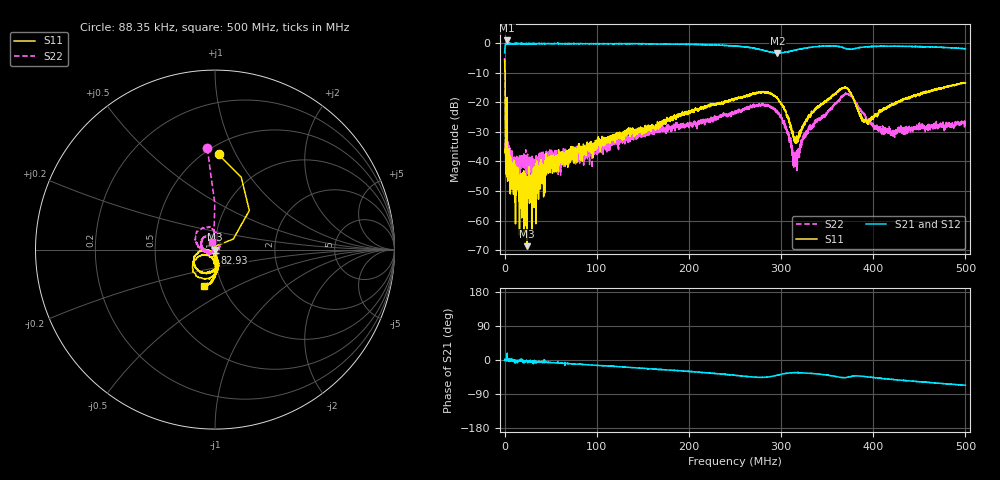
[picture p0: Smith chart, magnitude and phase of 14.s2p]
#  HZ  S  MA  R  50.00
! Rohde & Schwarz Vector Network Analyzer
! Rohde-Schwarz,ZNL6-2Port,1323001206101378,1.50.1.34-21.10.1.104
! Created: UTC 2/26/2024, 3:35:12 AM
! freq[Hz]  mag:S11  ang:S11  mag:S21  ang:S21  mag:S12  ang:S12  mag:S22  ang:S22
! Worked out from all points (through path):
!   5999 points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, 88.35 kHz to 500 MHz, reference 50 ohm
!   highest |S21| = 0.99 dB at 2.922 MHz (marker M1); lowest = -3.3 dB at 296.1 MHz (marker M2)
!   group delay of S21, straight-line fit = 332 ps
!   lowest |S11| = -68.7 dB at 24.34 MHz (marker M3), VSWR 1.00, Z = 50 - j0.0362 ohm
!   |S11| at or under -10 dB: 546.7 kHz to end of sweep
!   |S22| runs from -46.1 to -5.0 dB; largest |S21 - S12| = 0.35
!   S11 on the Smith chart (normalised r, x): 88.35 kHz: 0.58, +0.85; 82.93 MHz: 1.00, -0.04; 500 MHz: 0.82, -0.35
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88346.39  0.5305 87.8  0.6912 -1.2  0.6993 3.5  0.5653 94.3
2922124  0.1213 84.8  1.121 17.9  0.8209 7.2  0.1112 139.5
3838934  0.00873 145.6  0.9937 1.9  0.976 -2.9  0.01575 140.8
1.050665e7  0.005524 113.0  0.9865 -5.0  0.9874 1.7  0.009085 143.3
1.709101e7  0.002003 -136.5  0.9916 -1.8  0.988 -2.9  0.01002 166.5
2.434215e7  0.0003676 -79.9  0.9827 -4.1  0.9919 -2.5  0.01065 -176.5
4.634559e7  0.01126 -98.2  0.9913 -6.3  0.9911 -6.7  0.01222 -161.7
8.293466e7  0.01819 -84.7  0.9914 -11.5  0.9832 -12.3  0.0135 -145.4
8.343474e7  0.01502 -85.8  0.9844 -11.6  0.9895 -12.3  0.01474 -125.6
1.667811e8  0.03695 -87.1  0.971 -24.8  0.9789 -24.7  0.03512 -144.0
2.500442e8  0.1169 -91.8  0.9016 -40.2  0.9099 -40.5  0.06939 178.4
2.787987e8  0.1501 -126.3  0.7752 -46.0  0.7801 -45.3  0.09125 135.9
2.961347e8  0.1168 -161.1  0.6878 -39.9  0.6901 -39.1  0.06877 83.6
3.060529e8  0.06063 -178.4  0.7141 -34.9  0.7157 -34.5  0.03313 45.3
3.153044e8  0.0256 -143.7  0.7657 -33.2  0.7662 -32.9  0.01504 -58.3
3.240558e8  0.0391 -87.9  0.8224 -34.0  0.8204 -34.0  0.02187 -149.0
3.333906e8  0.06693 -78.2  0.8648 -35.3  0.8618 -36.1  0.03987 -162.0
3.717299e8  0.1732 -132.1  0.8062 -45.8  0.802 -48.3  0.1389 124.6
3.894827e8  0.04971 -140.5  0.8649 -43.3  0.8618 -45.1  0.06533 79.4
4.013179e8  0.06098 -101.1  0.8866 -46.3  0.8829 -48.4  0.03632 90.3
4.16737e8  0.08341 -87.5  0.8982 -50.2  0.8892 -52.7  0.02871 89.8
5e8  0.2149 -106.4  0.8124 -66.6  0.804 -69.2  0.04526 117.4
